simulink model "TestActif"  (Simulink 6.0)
settings: Solver=ode45  StartTime=0.0  StopTime=100  FixedStep=1E-3  RelTol=1e-3
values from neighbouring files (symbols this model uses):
  b = S/Sm    (= 0.1)    [Constantes.m]    (also in ConstantesBck.m)
  C = 1    [Constantes.m]    (also in ConstantesBck.m)
  Fact = 10^2    (= 100)    [Constantes.m]    (also in ConstantesBck.m)
  gk = 36    [Constantes.m]    (also in ConstantesBck.m; sim_hh.m)
  gl = 0.3    [Constantes.m]    (also in ConstantesBck.m; sim_hh.m)
  gna = 120    [Constantes.m]    (also in ConstantesBck.m; sim_hh.m)
  h0 = 0.5961    [Constantes.m]    (also in ConstantesBck.m)
  m0 = 0.0529    [Constantes.m]    (also in ConstantesBck.m)
  mK = 0    [Constantes.m]    (also in ConstantesBck.m)
  mL = 0    [Constantes.m]    (also in ConstantesBck.m)
  mNa = 0    [Constantes.m]    (also in ConstantesBck.m)
  n0 = 0.3177    [Constantes.m]    (also in ConstantesBck.m)
  Sm = 3.14e-2    (= 0.0314)    [Constantes.m]    (also in ConstantesBck.m = 0.000314)
  Vdd = 3.3*Rcan/Rct*1000    (= 3.2147881681)    [Constantes.m]    (also in ConstantesBck.m = 1.8)
  Vk = -82    [Constantes.m]    (also in ConstantesBck.m)
  Vl = -59    [Constantes.m]    (also in ConstantesBck.m)
  Vna = 45    [Constantes.m]    (also in ConstantesBck.m)
  Vr = -70    [Constantes.m]    (also in ConstantesBck.m)
libraries: simulink x2

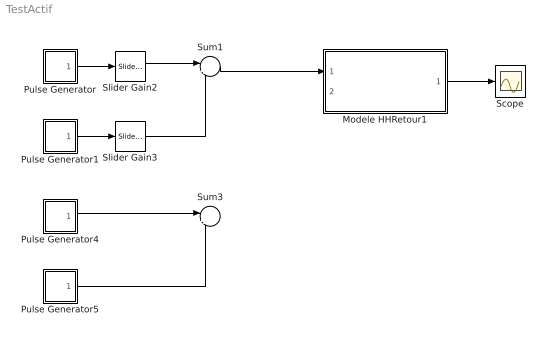
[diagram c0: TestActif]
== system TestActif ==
  Modele HHRetour1 : Subsystem
  Pulse Generator : Subsystem  mask(Pulse Generator){period=50, duty=4, amplitude=-1E-2, start=10}
      mask prompts: period "Period (secs):"; duty "Duty cycle (% of period):"; start "Start time:"
      mask help: Pulse Generator
  Pulse Generator1 : Subsystem  mask(Pulse Generator){period=50, duty=4, amplitude=1E-2, start=12}
      mask prompts: period "Period (secs):"; duty "Duty cycle (% of period):"; start "Start time:"
      mask help: Pulse Generator
  Pulse Generator4 : Subsystem  mask(Pulse Generator){period=50, duty=4, amplitude=Vdd, start=10}
      mask prompts: period "Period (secs):"; duty "Duty cycle (% of period):"; start "Start time:"
      mask help: Pulse Generator
  Pulse Generator5 : Subsystem  mask(Pulse Generator){period=50, duty=4, amplitude=-Vdd, start=14}
      mask prompts: period "Period (secs):"; duty "Duty cycle (% of period):"; start "Start time:"
      mask help: Pulse Generator
  Scope : Scope
  Slider Gain2 : simulink/Math Operations/Slider Gain  low=0  gain=36.406  high=100
  Slider Gain3 : simulink/Math Operations/Slider Gain  low=0  gain=43.779  high=100
  Sum1 : Sum  Inputs=|++
  Sum3 : Sum  Inputs=|++
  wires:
  Pulse Generator/1(out1) -> Slider Gain2/1
  Pulse Generator1/1(out1) -> Slider Gain3/1
  Slider Gain2/1 -> Sum1/1
  Slider Gain3/1 -> Sum1/2
  Pulse Generator4/1(out1) -> Sum3/1
  Pulse Generator5/1(out1) -> Sum3/2
  Modele HHRetour1/1(HHout) -> Scope/1
  Sum1/1 -> Modele HHRetour1/1(HHin)

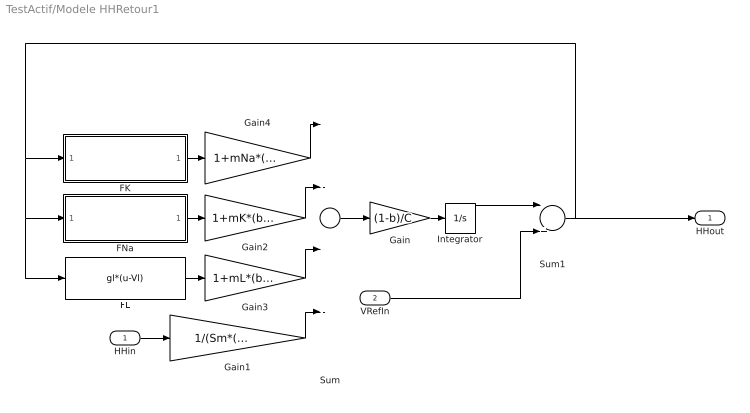
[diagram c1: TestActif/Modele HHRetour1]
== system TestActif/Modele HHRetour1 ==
  HHin : Inport  Port=1  LatchInput=off
  VRefIn : Inport  Port=2  LatchInput=off
  FK : Subsystem
  FL : Fcn  Expr=gl*(u-Vl)
  FNa : Subsystem
  Gain : Gain  Gain=(1-b)/C
  Gain1 : Gain  Gain=1/(Sm*(1-b)*Fact)
  Gain2 : Gain  Gain=1+mK*(b/(1-b))
  Gain3 : Gain  Gain=1+mL*(b/(1-b))
  Gain4 : Gain  Gain=1+mNa*(b/(1-b))
  Integrator : Integrator  InitialCondition=Vr
  Sum : Sum  Inputs=|---+
  Sum1 : Sum  Inputs=|++
  HHout : Outport
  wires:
  Sum/1 -> Gain/1
  Gain/1 -> Integrator/1
  FK/1(FKout) -> Gain4/1
  FNa/1(FNaOut) -> Gain2/1
  FL/1 -> Gain3/1
  HHin/1 -> Gain1/1
  Integrator/1 -> Sum1/1
  Sum1/1 -> FNa/1(FNaIn), FL/1, FK/1(FKIn), HHout/1
  Gain1/1 -> Sum/4
  Gain4/1 -> Sum/1
  Gain2/1 -> Sum/2
  Gain3/1 -> Sum/3
  VRefIn/1 -> Sum1/2

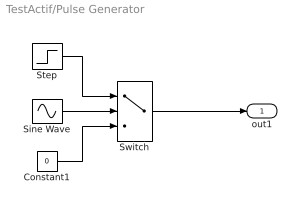
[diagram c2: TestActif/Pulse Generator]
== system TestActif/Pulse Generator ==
  Constant1 : Constant  Value=0
  Sine Wave : Sin  Frequency=2*pi./period  Phase=-2*pi*(start./period + duty/200 - 1/4)
  Step : Step  Time=start  After=amplitude
  Switch : Switch  Threshold=sin(pi*(0.5 - duty/100))
  out1 : Outport  InitialOutput=0
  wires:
  Step/1 -> Switch/1
  Constant1/1 -> Switch/3
  Switch/1 -> out1/1
  Sine Wave/1 -> Switch/2

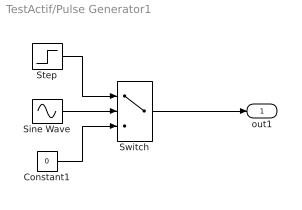
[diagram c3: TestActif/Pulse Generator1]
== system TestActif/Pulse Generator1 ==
  Constant1 : Constant  Value=0
  Sine Wave : Sin  Frequency=2*pi./period  Phase=-2*pi*(start./period + duty/200 - 1/4)
  Step : Step  Time=start  After=amplitude
  Switch : Switch  Threshold=sin(pi*(0.5 - duty/100))
  out1 : Outport  InitialOutput=0
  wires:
  Step/1 -> Switch/1
  Constant1/1 -> Switch/3
  Switch/1 -> out1/1
  Sine Wave/1 -> Switch/2

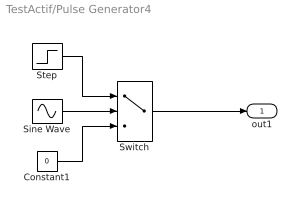
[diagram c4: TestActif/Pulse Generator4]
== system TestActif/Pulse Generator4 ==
  Constant1 : Constant  Value=0
  Sine Wave : Sin  Frequency=2*pi./period  Phase=-2*pi*(start./period + duty/200 - 1/4)
  Step : Step  Time=start  After=amplitude
  Switch : Switch  Threshold=sin(pi*(0.5 - duty/100))
  out1 : Outport  InitialOutput=0
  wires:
  Step/1 -> Switch/1
  Constant1/1 -> Switch/3
  Switch/1 -> out1/1
  Sine Wave/1 -> Switch/2

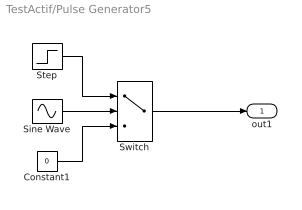
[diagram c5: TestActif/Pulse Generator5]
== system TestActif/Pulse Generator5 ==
  Constant1 : Constant  Value=0
  Sine Wave : Sin  Frequency=2*pi./period  Phase=-2*pi*(start./period + duty/200 - 1/4)
  Step : Step  Time=start  After=amplitude
  Switch : Switch  Threshold=sin(pi*(0.5 - duty/100))
  out1 : Outport  InitialOutput=0
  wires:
  Step/1 -> Switch/1
  Constant1/1 -> Switch/3
  Switch/1 -> out1/1
  Sine Wave/1 -> Switch/2

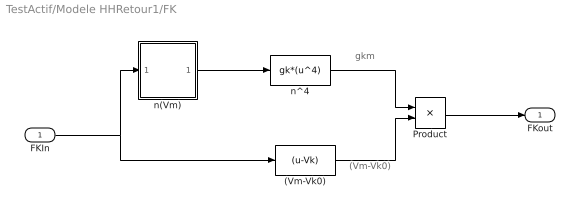
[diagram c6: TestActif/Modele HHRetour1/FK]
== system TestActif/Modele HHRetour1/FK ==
  note: gkm
  note: (Vm-Vk0)
  FKIn : Inport  Port=1  LatchInput=off
  (Vm-Vk0) : Fcn  Expr=(u-Vk)
  Product : Product
  n(Vm) : Subsystem
  n^4 : Fcn  Expr=gk*(u^4)
  FKout : Outport  InitialOutput=0
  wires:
  n(Vm)/1(n) -> n^4/1
  (Vm-Vk0)/1 -> Product/2
  Product/1 -> FKout/1
  n^4/1 -> Product/1
  FKIn/1 -> n(Vm)/1(Vm), (Vm-Vk0)/1

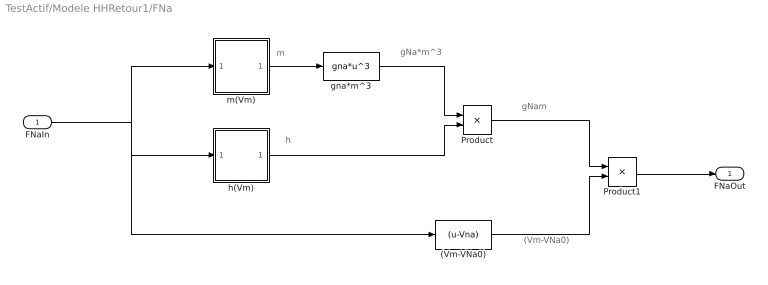
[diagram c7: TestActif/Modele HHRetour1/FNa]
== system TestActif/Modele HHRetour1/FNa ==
  note: gNa*m^3
  note: m
  note: h
  note: gNam
  note: (Vm-VNa0)
  FNaIn : Inport  Port=1  LatchInput=off
  (Vm-VNa0) : Fcn  Expr=(u-Vna)
  Product : Product
  Product1 : Product
  gna*m^3 : Fcn  Expr=gna*u^3
  h(Vm) : Subsystem
  m(Vm) : Subsystem
  FNaOut : Outport  InitialOutput=0
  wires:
  (Vm-VNa0)/1 -> Product1/2
  gna*m^3/1 -> Product/1
  Product1/1 -> FNaOut/1
  FNaIn/1 -> m(Vm)/1(Vm), h(Vm)/1(Vm), (Vm-VNa0)/1
  m(Vm)/1(n) -> gna*m^3/1
  h(Vm)/1(h) -> Product/2
  Product/1 -> Product1/1

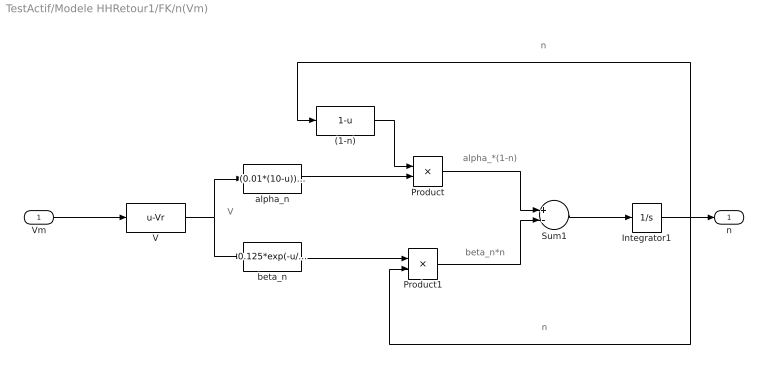
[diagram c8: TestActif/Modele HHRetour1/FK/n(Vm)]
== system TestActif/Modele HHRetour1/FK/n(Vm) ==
  note: V
  note: alpha_*(1-n)
  note: beta_n*n
  note: n
  note: n
  Vm : Inport  Port=1  LatchInput=off
  (1-n) : Fcn  Expr=1-u
  Integrator1 : Integrator  InitialCondition=n0
  Product : Product
  Product1 : Product
  Sum1 : Sum  Inputs=+-
  V : Fcn  Expr=u-Vr
  alpha_n : Fcn  Expr=(0.01*(10-u))/(exp((10-u)/10)-1)
  beta_n : Fcn  Expr=0.125*exp(-u/80)
  n : Outport  InitialOutput=0
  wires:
  V/1 -> alpha_n/1, beta_n/1
  alpha_n/1 -> Product/2
  (1-n)/1 -> Product/1
  beta_n/1 -> Product1/1
  Product/1 -> Sum1/1
  Product1/1 -> Sum1/2
  Sum1/1 -> Integrator1/1
  Integrator1/1 -> (1-n)/1, Product1/2, n/1
  Vm/1 -> V/1

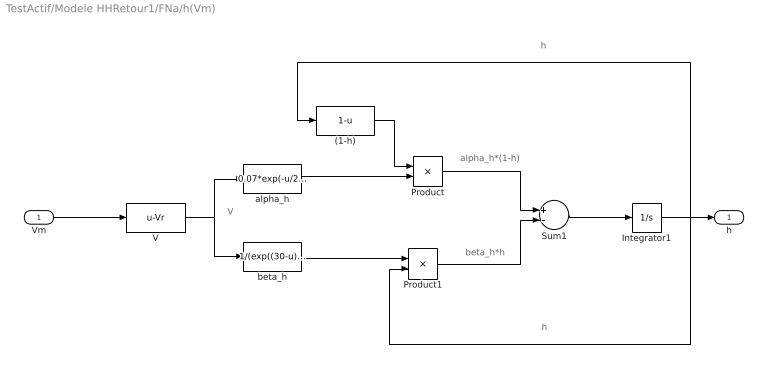
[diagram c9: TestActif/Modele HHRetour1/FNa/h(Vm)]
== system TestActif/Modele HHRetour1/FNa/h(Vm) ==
  note: h
  note: h
  note: beta_h*h
  note: alpha_h*(1-h)
  note: V
  Vm : Inport  Port=1  LatchInput=off
  (1-h) : Fcn  Expr=1-u
  Integrator1 : Integrator  InitialCondition=h0
  Product : Product
  Product1 : Product
  Sum1 : Sum  Inputs=+-
  V : Fcn  Expr=u-Vr
  alpha_h : Fcn  Expr=0.07*exp(-u/20)
  beta_h : Fcn  Expr=1/(exp((30-u)/10)+1)
  h : Outport  InitialOutput=0
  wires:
  Vm/1 -> V/1
  Integrator1/1 -> h/1, Product1/2, (1-h)/1
  Sum1/1 -> Integrator1/1
  Product1/1 -> Sum1/2
  Product/1 -> Sum1/1
  beta_h/1 -> Product1/1
  (1-h)/1 -> Product/1
  alpha_h/1 -> Product/2
  V/1 -> beta_h/1, alpha_h/1

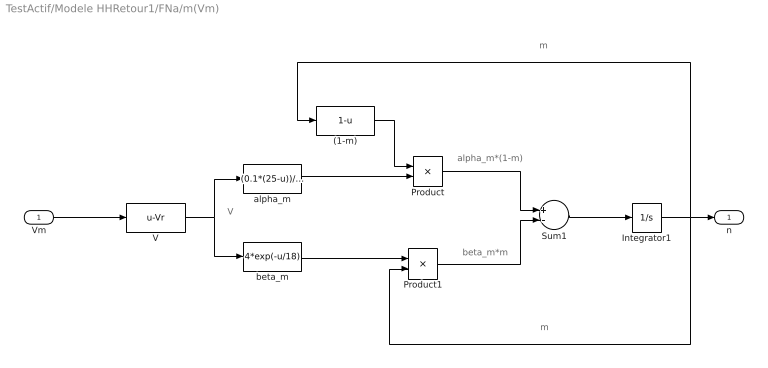
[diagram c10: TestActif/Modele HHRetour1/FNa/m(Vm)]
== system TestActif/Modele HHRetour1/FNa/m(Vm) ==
  note: m
  note: m
  note: beta_m*m
  note: alpha_m*(1-m)
  note: V
  Vm : Inport  Port=1  LatchInput=off
  (1-m) : Fcn  Expr=1-u
  Integrator1 : Integrator  InitialCondition=m0
  Product : Product
  Product1 : Product
  Sum1 : Sum  Inputs=+-
  V : Fcn  Expr=u-Vr
  alpha_m : Fcn  Expr=(0.1*(25-u))/(exp((25-u)/10)-1)
  beta_m : Fcn  Expr=4*exp(-u/18)
  n : Outport  InitialOutput=0
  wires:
  Vm/1 -> V/1
  Integrator1/1 -> n/1, Product1/2, (1-m)/1
  Sum1/1 -> Integrator1/1
  Product1/1 -> Sum1/2
  Product/1 -> Sum1/1
  beta_m/1 -> Product1/1
  (1-m)/1 -> Product/1
  alpha_m/1 -> Product/2
  V/1 -> beta_m/1, alpha_m/1
